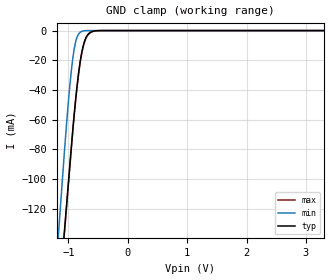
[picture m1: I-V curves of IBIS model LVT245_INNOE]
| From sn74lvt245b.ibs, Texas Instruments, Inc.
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[Model]   LVT245_INNOE
Model_type  Input
Vinl=0.8
Vinh=2.0
| variable   typ   min   max
C_comp   4.27pF   3.18pF   5.53pF
[Temperature Range]   40   -40   100
| Ambient temperature   25   -40   85
[Voltage range]   3.3   2.7   3.6
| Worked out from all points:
|   GND clamp passes 1 mA (typ) near -0.62 V on its own axis
[GND Clamp]
| LVT245_INNOE
|   Voltage   I(typ)   I(min)   I(max)
-5.5V     -2.756A    -2.979A    -2.783A
-1.17V    -185.1mA   -138.6mA   -189.6mA
-1.14V    -170.5mA   -121.9mA   -174mA
-1.075V   -138.9mA   -85.8mA    -140.9mA
-1.05V    -126.7mA   -72.62mA   -128.3mA
-975mV    -90.31mA   -36.58mA   -91.26mA
-900mV    -55.41mA   -11.77mA   -56.15mA
-825mV    -27.54mA   -2.142mA   -28.17mA
-775mV    -14.76mA   -541.2uA   -15.31mA
-725mV    -6.791mA   -95.21uA   -7.264mA
-650mV    -1.754mA   -6.225uA   -2.087mA
3.3V      29.99pA    22.28pA    2.568nA
